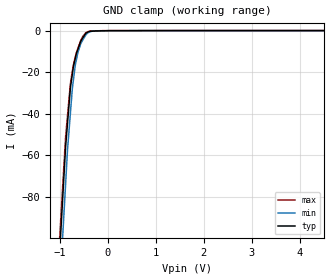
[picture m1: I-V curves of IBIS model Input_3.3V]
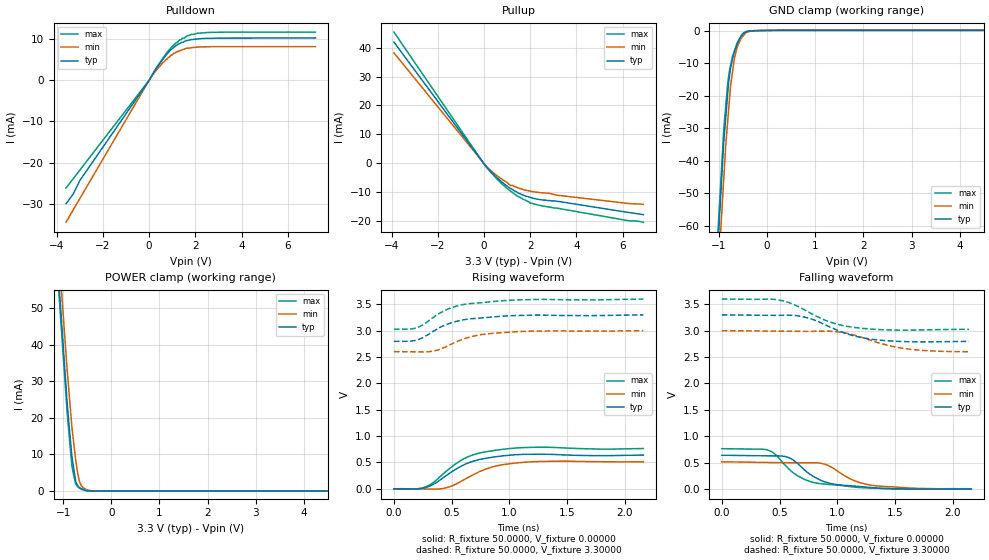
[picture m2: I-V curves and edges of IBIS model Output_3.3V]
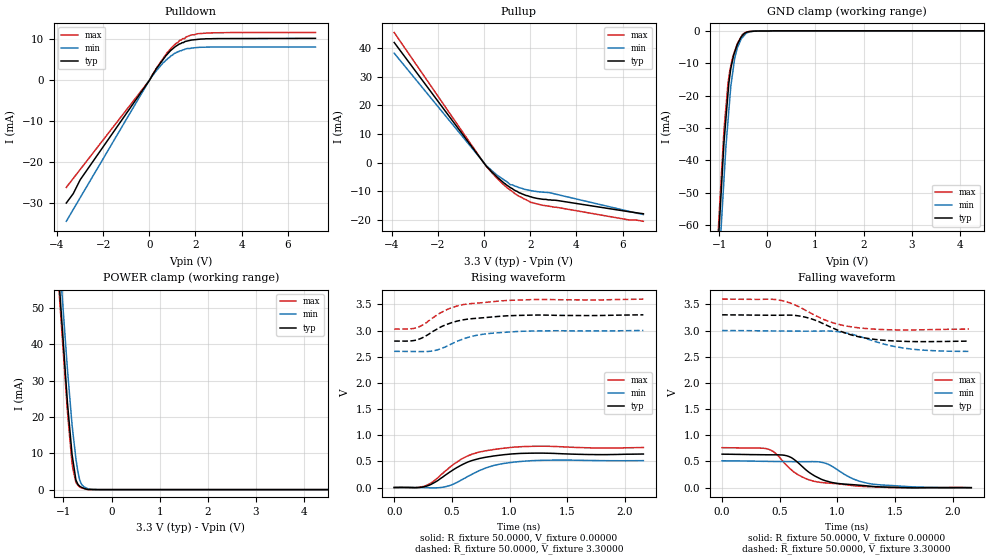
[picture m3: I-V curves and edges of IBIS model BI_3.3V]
[IBIS Ver]   3.2
[Comment Char] |_char
[File Name]   pcm1802db.ibs
[File Rev]   3.0
[Source]
| This model file was created by Teraspeed Consulting Group LLC
| (http://www.teraspeed.com/).
[Date]   08-19-2004
[Notes]   Quality Check of this IBIS model: Model Passes IBIS Check
   Model parses into ICX IS. Simulation done with Hyperlynx.
   1. MIN TYP MAX information is based on Temprature and Voltage
   characteristics only.
[Disclaimer]
| This model is designed as an aid for customers of Texas Instruments.
| TI and its licensors and suppliers make no warranties, either expressed
| or implied, with respect to this  model, including the warranties of
| merchantability or fitness for a particular purpose.
| The model is provided solely on an "as is" basis. The entire risk as to
| its quality and performance is with the customer.
[Copyright]
| (C) Copyright 2008 Texas Instruments Incorporated. All rights reserved.
[Component] PCM1802DB
[Manufacturer] TI
[Package]
| variable   typ   min   max
R_pkg  1.7363E-02  1.7363E-02  1.7363E-02
L_pkg  2.1878E-09  2.1878E-09  2.1878E-09
C_pkg  4.4649E-13  4.4649E-13  4.4649E-13
[Pin] signal_name  model_name  R_pin  L_pin C_pin
1   VinL   Input_3.3V   1.9723E-02  2.4851E-09  5.0716E-13
2   VinR   Input_3.3V   1.8868E-02  2.3774E-09  4.8518E-13
3   Vref1  POWER   1.8028E-02  2.2715E-09  4.6357E-13
4   Vref2  POWER   1.7205E-02  2.1678E-09  4.4241E-13
5   Vcc   POWER   1.6401E-02  2.0666E-09  4.2175E-13
6   AGND   GND   1.5620E-02  1.9682E-09  4.0167E-13
7   _PDWN  Input_3.3V   1.4866E-02  1.8731E-09  3.8227E-13
8   BYPAS  Input_3.3V   1.4866E-02  1.8731E-09  3.8227E-13
9   FSYNC  BI_3.3V   1.5620E-02  1.9682E-09  4.0167E-13
10  LRCK   BI_3.3V   1.6401E-02  2.0666E-09  4.2175E-13
11  BCK   BI_3.3V   1.7205E-02  2.1678E-09  4.4241E-13
12  DOUT   Output_3.3V  1.8028E-02  2.2715E-09  4.6357E-13
13  DGND   GND   1.8868E-02  2.3774E-09  4.8518E-13
14  Vdd   POWER   1.9723E-02  2.4851E-09  5.0716E-13
15  SCKI   Input_3.3V   1.9723E-02  2.4851E-09  5.0716E-13
16  OSR   Input_3.3V   1.8868E-02  2.3774E-09  4.8518E-13
17  FMT0   Input_3.3V   1.8028E-02  2.2715E-09  4.6357E-13
18  FMT1   Input_3.3V   1.7205E-02  2.1678E-09  4.4241E-13
19  MODE0  Input_3.3V   1.6401E-02  2.0666E-09  4.2175E-13
20  MODE1  Input_3.3V   1.5620E-02  1.9682E-09  4.0167E-13
| Models and submodels in the file (3): Input_3.3V (Input), Output_3.3V (Output), BI_3.3V (Output)
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[Model] Input_3.3V
Model_type Input
Vinl  = 800.000mV
Vinh  = 2.00000V
C_comp  2.00000pF 2.00000pF 2.00000pF
| variable   typ   min   max
[Voltage Range]   3.30000V  3.00000V  3.60000V
[POWER Clamp Reference]  3.30000V  3.00000V  3.60000V
[GND Clamp Reference]   0.00000V  0.00000V  0.00000V
[Temperature Range]   25   85   -25
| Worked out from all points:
|   GND clamp passes 1 mA (typ) near -0.45 V on its own axis
[GND Clamp]
-3.3V     -1.046A    -1.078A    -999.8mA
-881mV    -55.89mA   -73.94mA   -51.06mA
-840.9mV  -44.51mA   -57.27mA   -40.77mA
-780.3mV  -27.35mA   -39.56mA   -25.27mA
-739.7mV  -20.7mA    -27.67mA   -19.41mA
-719.4mV  -17.38mA   -23.97mA   -16.48mA
-679.1mV  -13.22mA   -16.6mA    -12.61mA
-623.4mV  -8.829mA   -10.38mA   -8.374mA
-562.1mV  -4.848mA   -6.036mA   -4.405mA
-420.8mV  -625.3uA   -1.071mA   -442.3uA
61.63mV   65.1uA     47.55uA    79.25uA
6.6V      102.1uA    79.84uA    108.8uA
[POWER Clamp]
| Voltage   I(typ)   I(min)   I(max)
-3.6V     0A         0A         0A
-3.5V     0A         0A         0A
-3.4V     0A         0A         0A
7.2V      0A         0A         0A
[Model] Output_3.3V
Model_type Output
Vref  = 0.00000V
Cref  = 2.00000pF
Vmeas = 1.65000V
C_comp  2.00000pF 2.00000pF 2.00000pF
| variable   typ   min   max
[Voltage Range]   3.30000V  3.00000V  3.60000V
[POWER Clamp Reference]  3.30000V  3.00000V  3.60000V
[Pullup Reference]   3.30000V  3.00000V  3.60000V
[Pulldown Reference]   0.00000V  0.00000V  0.00000V
[GND Clamp Reference]   0.00000V  0.00000V  0.00000V
[Temperature Range]   25   85   -25
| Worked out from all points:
|   slope of the pulldown table from 0 to 0.495 V, typ, clamps not added: 114 ohm
|   slope of the pullup table from 0 to 0.495 V, typ, clamps not added: 115 ohm
|   GND clamp passes 1 mA (typ) near -0.49 V on its own axis
|   POWER clamp passes 1 mA (typ) near -0.67 V on its own axis
|   rising waveform, R_fixture 50.0000, V_fixture 0.00000: 20-80 % time 296ps typ, 298ps min, 286ps max; typ from 0 V to 0.64 V
|   falling waveform, R_fixture 50.0000, V_fixture 0.00000: 20-80 % time 263ps typ, 275ps min, 265ps max; typ from 0.64 V to 0 V
|   falling waveform, R_fixture 50.0000, V_fixture 3.30000: 20-80 % time 347ps typ, 388ps min, 335ps max; typ from 3.3 V to 2.8 V
|   rising waveform, R_fixture 50.0000, V_fixture 3.30000: 20-80 % time 312ps typ, 307ps min, 303ps max; typ from 2.8 V to 3.3 V
[GND Clamp]
-3.3V     -663.9mA   -649.4mA   -654.5mA
-901.3mV  -34.29mA   -45.71mA   -30.48mA
-861mV    -27mA      -35.59mA   -23.51mA
-820.7mV  -19.68mA   -28.2mA    -16.52mA
-800.4mV  -15.99mA   -24.47mA   -14.33mA
-760mV    -11.56mA   -17.07mA   -10.77mA
-679.1mV  -6.503mA   -8.377mA   -6.246mA
-623.5mV  -4.109mA   -5.157mA   -3.867mA
-542.3mV  -1.775mA   -2.401mA   -1.705mA
-420.8mV  -320.8uA   -560.4uA   -245.7uA
219mV     59.07uA    63.58uA    60.52uA
6.6V      59.47uA    63.58uA    67.83uA
[Pulldown]
-3.6V     -29.93mA   -34.38mA   -26.13mA
-3.3V     -27.66mA   -31.52mA   -23.96mA
-3V       -24.3mA    -28.66mA   -21.79mA
20.8mV    92.19uA    132.4uA    70.78uA
299.7mV   2.737mA    2.231mA    2.811mA
800.2mV   6.424mA    5.253mA    6.883mA
941.6mV   7.269mA    5.945mA    7.724mA
1.179V    8.327mA    6.76mA     9.042mA
1.442V    9.105mA    7.336mA    10.09mA
2.079V    9.887mA    7.918mA    11.27mA
3.499V    10.1mA     8.032mA    11.56mA
7.2V      10.15mA    8.034mA    11.56mA
[Pullup]
-3.9V     41.97mA    38.24mA    45.43mA
0V        -205.8uA   -93.41uA   -224.9uA
558.8mV   -4.994mA   -4.304mA   -5.448mA
1.059V    -8.264mA   -7.135mA   -9.128mA
1.14V     -8.721mA   -7.709mA   -9.591mA
1.241V    -9.166mA   -7.715mA   -10.17mA
1.55V     -10.59mA   -8.771mA   -11.83mA
2.02V     -11.9mA    -9.713mA   -13.9mA
2.56V     -12.77mA   -10.29mA   -14.89mA
3.178V    -13.19mA   -11.11mA   -15.6mA
6.3V      -17.13mA   -14mA      -19.99mA
6.9V      -17.8mA    -14.27mA   -20.44mA
[POWER Clamp]
-3.3V     482.3mA    472.9mA    476.2mA
-1.12V    62.92mA    70.53mA    60.14mA
-1.059V   51.29mA    59.37mA    48.59mA
-1.019V   43.5mA     51.9mA     40.87mA
-917.8mV  24.11mA    33.29mA    21.63mA
-821.6mV  9.739mA    17.94mA    7.222mA
-740.9mV  2.661mA    8.489mA    1.999mA
-700.4mV  1.478mA    4.98mA     1.206mA
-659.8mV  903.6uA    2.513mA    708.6uA
-619.5mV  579.5uA    1.379mA    436.6uA
-381.6mV  25.51uA    2.953uA    5.591uA
6.6V      0A         0A         0A
[Rising Waveform]
R_fixture = 50.0000
V_fixture = 0.00000
V_fixture_min = 0.00000
V_fixture_max = 0.00000
0s        0V         0V         0V
200ps     -1.756mV   -1.29mV    661.3uV
280ps     26.15mV    -4.339mV   41.27mV
440ps     231.4mV    13.26mV    310.4mV
580ps     426.2mV    140.6mV    540.1mV
680ps     519.2mV    259.8mV    641.3mV
800ps     580.7mV    378mV      704.2mV
940ps     623.8mV    456.2mV    748.6mV
1.2ns     656.1mV    513.4mV    786.9mV
2.16ns    639.8mV    513.2mV    763.8mV
[Falling Waveform]
R_fixture = 50.0000
V_fixture = 0.00000
V_fixture_min = 0.00000
V_fixture_max = 0.00000
0s        639.8mV    513.2mV    763.8mV
400ps     627.7mV    501.8mV    735.6mV
460ps     627.3mV    500.2mV    661.9mV
580ps     594.4mV    497.7mV    379.7mV
700ps     392.8mV    496.6mV    198.2mV
820ps     204mV      496.3mV    112.1mV
980ps     88.21mV    370.3mV    77.85mV
1.14ns    55.86mV    164mV      38.02mV
1.28ns    28.97mV    76.56mV    18.09mV
2.16ns    0V         0V         0V
[Falling Waveform]
R_fixture = 50.0000
V_fixture = 3.30000
V_fixture_min = 3.00000
V_fixture_max = 3.60000
0s        3.3V       3V         3.6V
460ps     3.292V     2.992V     3.592V
560ps     3.295V     2.99V      3.547V
680ps     3.274V     2.989V     3.439V
780ps     3.219V     2.988V     3.319V
920ps     3.087V     2.991V     3.178V
1.18ns    2.884V     2.897V     3.053V
1.4ns     2.815V     2.743V     3.019V
1.58ns    2.793V     2.664V     3.011V
2.14ns    2.798V     2.602V     3.027V
[Rising Waveform]
R_fixture = 50.0000
V_fixture = 3.30000
V_fixture_min = 3.00000
V_fixture_max = 3.60000
0s        2.798V     2.602V     3.027V
120ps     2.799V     2.6V       3.029V
200ps     2.823V     2.598V     3.057V
260ps     2.879V     2.598V     3.122V
340ps     2.989V     2.613V     3.25V
480ps     3.136V     2.726V     3.421V
640ps     3.218V     2.868V     3.509V
800ps     3.249V     2.938V     3.54V
1.12ns    3.291V     2.987V     3.586V
2.16ns    3.3V       3V         3.6V
[Ramp]
| variable  typ   min   max
dV/dt_r   381.416m/420.508p  306.230m/472.835p  454.372m/391.970p
dV/dt_f   306.377m/426.304p  242.479m/473.539p  349.654m/394.914p
R_load = 50.0000Ohms
[Model] BI_3.3V
Model_type Output
Vref  = 0.00000V
Cref  = 2.00000pF
Vmeas = 1.65000V
C_comp  2.00000pF 2.00000pF 2.00000pF
| variable   typ   min   max
[Voltage Range]   3.30000V  3.00000V  3.60000V
[POWER Clamp Reference]  3.30000V  3.00000V  3.60000V
[Pullup Reference]   3.30000V  3.00000V  3.60000V
[Pulldown Reference]   0.00000V  0.00000V  0.00000V
[GND Clamp Reference]   0.00000V  0.00000V  0.00000V
[Temperature Range]   25   85   -25
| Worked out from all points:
|   slope of the pulldown table from 0 to 0.495 V, typ, clamps not added: 114 ohm
|   slope of the pullup table from 0 to 0.495 V, typ, clamps not added: 115 ohm
|   GND clamp passes 1 mA (typ) near -0.49 V on its own axis
|   POWER clamp passes 1 mA (typ) near -0.67 V on its own axis
|   rising waveform, R_fixture 50.0000, V_fixture 0.00000: 20-80 % time 296ps typ, 298ps min, 286ps max; typ from 0 V to 0.64 V
|   falling waveform, R_fixture 50.0000, V_fixture 0.00000: 20-80 % time 263ps typ, 275ps min, 265ps max; typ from 0.64 V to 0 V
|   falling waveform, R_fixture 50.0000, V_fixture 3.30000: 20-80 % time 347ps typ, 388ps min, 335ps max; typ from 3.3 V to 2.8 V
|   rising waveform, R_fixture 50.0000, V_fixture 3.30000: 20-80 % time 312ps typ, 307ps min, 303ps max; typ from 2.8 V to 3.3 V
[GND Clamp]
-3.3V     -663.9mA   -649.4mA   -654.5mA
-901.3mV  -34.29mA   -45.71mA   -30.48mA
-861mV    -27mA      -35.59mA   -23.51mA
-820.7mV  -19.68mA   -28.2mA    -16.52mA
-800.4mV  -15.99mA   -24.47mA   -14.33mA
-760mV    -11.56mA   -17.07mA   -10.77mA
-679.1mV  -6.503mA   -8.377mA   -6.246mA
-623.5mV  -4.109mA   -5.157mA   -3.867mA
-542.3mV  -1.775mA   -2.401mA   -1.705mA
-420.8mV  -320.8uA   -560.4uA   -245.7uA
219mV     59.07uA    63.58uA    60.52uA
6.6V      59.47uA    63.58uA    67.83uA
[Pulldown]
-3.6V     -29.93mA   -34.38mA   -26.13mA
-3.3V     -27.66mA   -31.52mA   -23.96mA
-3V       -24.3mA    -28.66mA   -21.79mA
20.8mV    92.19uA    132.4uA    70.78uA
299.7mV   2.737mA    2.231mA    2.811mA
800.2mV   6.424mA    5.253mA    6.883mA
941.6mV   7.269mA    5.945mA    7.724mA
1.179V    8.327mA    6.76mA     9.042mA
1.442V    9.105mA    7.336mA    10.09mA
2.079V    9.887mA    7.918mA    11.27mA
3.499V    10.1mA     8.032mA    11.56mA
7.2V      10.15mA    8.034mA    11.56mA
[Pullup]
-3.9V     41.97mA    38.24mA    45.43mA
0V        -205.8uA   -93.41uA   -224.9uA
98.2mV    -1.268mA   -1.059mA   -1.291mA
558.8mV   -4.994mA   -4.304mA   -5.448mA
1.059V    -8.264mA   -7.135mA   -9.128mA
1.14V     -8.721mA   -7.709mA   -9.591mA
1.241V    -9.166mA   -7.715mA   -10.17mA
1.55V     -10.59mA   -8.771mA   -11.83mA
2.02V     -11.9mA    -9.713mA   -13.9mA
2.879V    -12.96mA   -10.52mA   -15.25mA
6.3V      -17.13mA   -17mA      -19.99mA
6.9V      -17.8mA    -18.07mA   -20.44mA
[POWER Clamp]
-3.3V     482.3mA    472.9mA    476.2mA
-1.12V    62.92mA    70.53mA    60.14mA
-1.059V   51.29mA    59.37mA    48.59mA
-1.019V   43.5mA     51.9mA     40.87mA
-917.8mV  24.11mA    33.29mA    21.63mA
-821.6mV  9.739mA    17.94mA    7.222mA
-740.9mV  2.661mA    8.489mA    1.999mA
-700.4mV  1.478mA    4.98mA     1.206mA
-659.8mV  903.6uA    2.513mA    708.6uA
-619.5mV  579.5uA    1.379mA    436.6uA
-381.6mV  25.51uA    2.953uA    5.591uA
6.6V      0A         0A         0A
[Rising Waveform]
R_fixture = 50.0000
V_fixture = 0.00000
V_fixture_min = 0.00000
V_fixture_max = 0.00000
0s        0V         0V         0V
200ps     -1.756mV   -1.29mV    661.3uV
280ps     26.15mV    -4.339mV   41.27mV
440ps     231.4mV    13.26mV    310.4mV
580ps     426.2mV    140.6mV    540.1mV
680ps     519.2mV    259.8mV    641.3mV
800ps     580.7mV    378mV      704.2mV
940ps     623.8mV    456.2mV    748.6mV
1.2ns     656.1mV    513.4mV    786.9mV
2.16ns    639.8mV    513.2mV    763.8mV
[Falling Waveform]
R_fixture = 50.0000
V_fixture = 0.00000
V_fixture_min = 0.00000
V_fixture_max = 0.00000
0s        639.8mV    513.2mV    763.8mV
400ps     627.7mV    501.8mV    735.6mV
460ps     627.3mV    500.2mV    661.9mV
580ps     594.4mV    497.7mV    379.7mV
700ps     392.8mV    496.6mV    198.2mV
820ps     204mV      496.3mV    112.1mV
980ps     88.21mV    370.3mV    77.85mV
1.14ns    55.86mV    164mV      38.02mV
1.28ns    28.97mV    76.56mV    18.09mV
2.16ns    0V         0V         0V
[Falling Waveform]
R_fixture = 50.0000
V_fixture = 3.30000
V_fixture_min = 3.00000
V_fixture_max = 3.60000
0s        3.3V       3V         3.6V
460ps     3.292V     2.992V     3.592V
560ps     3.295V     2.99V      3.547V
680ps     3.274V     2.989V     3.439V
780ps     3.219V     2.988V     3.319V
920ps     3.087V     2.991V     3.178V
1.18ns    2.884V     2.897V     3.053V
1.4ns     2.815V     2.743V     3.019V
1.58ns    2.793V     2.664V     3.011V
2.14ns    2.798V     2.602V     3.027V
[Rising Waveform]
R_fixture = 50.0000
V_fixture = 3.30000
V_fixture_min = 3.00000
V_fixture_max = 3.60000
0s        2.798V     2.602V     3.027V
120ps     2.799V     2.6V       3.029V
200ps     2.823V     2.598V     3.057V
260ps     2.879V     2.598V     3.122V
340ps     2.989V     2.613V     3.25V
480ps     3.136V     2.726V     3.421V
640ps     3.218V     2.868V     3.509V
800ps     3.249V     2.938V     3.54V
1.12ns    3.291V     2.987V     3.586V
2.16ns    3.3V       3V         3.6V
[Ramp]
| variable  typ   min   max
dV/dt_r   381.416m/420.508p  306.230m/472.835p  454.372m/391.970p
dV/dt_f   306.377m/426.304p  242.479m/473.539p  349.654m/394.914p
R_load = 50.0000Ohms
